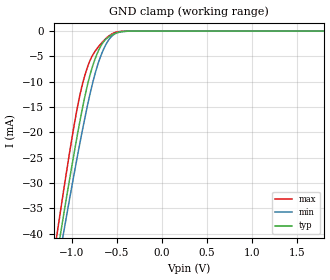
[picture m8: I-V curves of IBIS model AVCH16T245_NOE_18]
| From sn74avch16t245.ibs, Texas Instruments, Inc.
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[Model]   AVCH16T245_NOE_18
Model_type  Input
Vinl=0.5775
Vinh=1.2675
| variable   typ   min   max
C_comp   2.93pF   2.38pF   3.43pF
[Temperature Range]   40   100   -40
| Ambient temperature   25   85   -40
[Voltage range]   1.8   1.65   1.95
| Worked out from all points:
|   GND clamp passes 1 mA (typ) near -0.58 V on its own axis
[GND Clamp]
| AVCH16T245_NOE_18
|   Voltage   I(typ)   I(min)   I(max)
-4.6V     -463.5mA   -440.8mA   -490.1mA
-1.185V   -46.55mA   -49.44mA   -42.56mA
-1.155V   -43.24mA   -46.33mA   -38.98mA
-1.13V    -40.5mA    -43.76mA   -36.02mA
-1.105V   -37.79mA   -41.2mA    -33.1mA
-1.08V    -35.1mA    -38.66mA   -30.2mA
-950mV    -21.65mA   -25.86mA   -16.19mA
-840mV    -11.71mA   -15.87mA   -7.878mA
-765mV    -6.713mA   -9.994mA   -4.647mA
-690mV    -3.355mA   -5.483mA   -2.782mA
-535mV    -575.1uA   -706uA     -397.6uA
1.8V      159.1pA    895pA      30.75pA
